// TwinCAT 3 PLC project UPS_IPC_test
// ProgramVersion: 3.1.4023.0
// libraries:
//   Tc2_Standard, * (Beckhoff Automation GmbH)
//   Tc2_System, * (Beckhoff Automation GmbH)
//   Tc2_Utilities, * (Beckhoff Automation GmbH)
//   Tc3_Module, * (Beckhoff Automation GmbH)
// project tree:
//   / PlcTask.TcTTO
//   POUs/ MAIN.TcPOU
// real-time tasks:
//   TASK PlcTask: cycle T#10ms, priority 20, ADS port 350

CONFIGURATION UPS_IPC_test
    RESOURCE PLC ON TwinCAT3
        TASK PlcTask(INTERVAL := T#10ms, PRIORITY := 20);
        PROGRAM MAIN WITH PlcTask : MAIN;
    END_RESOURCE
END_CONFIGURATION

// ---- POUs/MAIN.TcPOU
PROGRAM MAIN
VAR
	b_pfail AT %I*: BOOL;								//用于接收CU8110-0120的P FAIL口输出的关闭Uin的输入电压
	b_upsen AT %Q*: BOOL:= TRUE;						//用于给CU8110-0120的UPS EN	口输入高电平，当P Fail口有输出时给UPS EN口一个下降沿用于关闭U1,2out的输出
	b_upsready AT %I*:BOOL;
	FB_WritePersistentData: FB_WritePersistentData;		//该功能块用于写入持续的数据起到掉电数据保存的功能
	b_start: BOOL;
	b_busy: BOOL;
	FB_TON: TON;
	b_PSHDN AT %Q*: BOOL;
END_VAR
VAR PERSISTENT
	Array_persistent: ARRAY[0..1048575] OF byte;
END_VAR

FB_WritePersistentData(
	NETID:= , 							//默认为本地的NetId,功能块会自动获取
	PORT:= 851, 						//输入PLC运行时系统的端口号，此处为851
	START:= b_start, 					//触发引脚，触发写入PersistentData并储存		
	TMOUT:= , 
	MODE:= , 							//默认为Persistent数据的写入模式:SPDM_2PASS
	BUSY=> b_busy, 						//输出功能块的运行状态
	ERR=> , 
	ERRID=> );
FB_TON(IN:= , PT:=T#2S , Q=> , ET=> );	//用于延迟2s给b_upsen一个下降沿以确保PersistentData存储完毕
IF b_pfail=TRUE THEN					//当检测到关闭Uin的输入电压时
	b_start:=TRUE;						//触发FB_WritePersistentData功能块开始写入并储存PersistentData
	IF NOT(b_busy=TRUE) THEN			//当储存完毕后
			FB_TON.IN:=TRUE;			//触发TON功能块
			IF FB_TON.Q=TRUE THEN		//当设定时间2s后
				b_upsen:=FALSE;			//给b_upsen下降沿信号用于关闭U1,2out口的输出完成关闭所连接的工控机
			END_IF
	END_IF
ELSE
	b_upsen:=TRUE;						//若没有检测到关闭Uin的输入电压时b_upsen保持高电平
END_IF

END_PROGRAM
